(* Logix 5000 AddOnInstructionDefinition export Process_TU3VFDControl_Instance100_101; software revision 24.02 *)

TYPE FI_Data_IN :
STRUCT
   ConnectionFaulted : BOOL;
   RunMode : BOOL;
   Data : INT[6];   // Actual Values
END_STRUCT
END_TYPE

TYPE FI_Data_OUT :
STRUCT
   Data : INT[6];   // Control Data
END_STRUCT
END_TYPE

ADD_ON_INSTRUCTION Process_TU3VFDControl_Instance100_101   (* revision 1.1, vendor NORD Drivesystems, ExecutePrescan *)
// Control block for Nord VFD TU3 Instances 100/101
// Allows for control of one (1) SK 5xxE VFD.
// Revision note:
// Rev 1.1
// Better Ready Start Condition Logic
// Added Inhibited Output
// Added Fault Active Output
// Rev 1.0
VAR_IN_OUT
   FI_Status : _0342:TU3_EIP_DE5BFA94:I:0; {required}   // Input Data Map of VFD
   FI_Control : _0342:TU3_EIP_E8E6FFA2:O:0; {required}   // Output Data Map of VFD
END_VAR
VAR_INPUT
   VFD_Number : SINT := 1;   // Number of VFD to control (1 for Instance 100/101)
   EnableFwd : BOOL; {visible}   // HIGH = Enable CW
   EnableRev : BOOL; {visible}   // HIGH = Enable CCW
   DisableVoltage : BOOL := 1; {visible}   // LOW = No Output Voltage
   QuickStop : BOOL := 1; {visible}   // LOW = Emergency Stop Active
   FaultAckn : BOOL; {visible}   // Error / Fault Acknowledgement on Rising Edge
   ParameterSet : SINT; {visible}   // Parameter Set 1-4, If less than 1 or higher than 4, Set 1 as active
   Activate32BitSetpoint : BOOL; {visible}   // HIGH = Activate 32Bit Setpoint combining Setpoint 2 & 3
   ControlWordBit8_P480_11 : BOOL; {visible}   // Control Word Bit 8 Function set in P480[11]
   ControlWordBit9_P480_12 : BOOL; {visible}   // Control Word Bit 9 Function set in P480[12]
END_VAR
VAR_OUTPUT
   ControlWord : ALIAS FOR Control_Word; {access Read Only, visible}   // Control Word Read Only Version
END_VAR
VAR_INPUT
   Setpoint1 : INT; {visible}   // Setpoint 1 Function set in P546
   Setpoint2 : INT; {visible}   // Setpoint 2 Function set in P547, deactivated if "PositioningActiveBit" is set
   Setpoint3 : INT; {visible}   // Setpoint 3 Function set in P548, deactivated if "PositioningActiveBitt" is set
   Setpoint4 : INT;   // Setpoint 4 Only available in SK 54xE
   Setpoint5 : INT;   // Setpoint 5 Only available in SK 54xE
   Setpoint2_3_32 : DINT; {visible}   // 32 Bit Setpoint 2 & 3 combined for positioning
END_VAR
VAR_OUTPUT
   StatusWord : INT; {access Read Only, visible}   // Status Word
        .0   // Ready to Start
        .1   // Ready for Operation
        .2   // Operation Enabled
        .3   // Fault
        .4   // Voltage Enabled
        .5   // No Emergency Stop
        .6   // Starting Disabled
        .7   // Warning Active
        .8   // Setpoint Reached
        .9   // Bus Controller Active
        .10   // Function P481[9]
        .11   // Rotation Right Active
        .12   // Rotation Left Active
        .13   // Function P481[10]
        .14   // Parameter Set Bit 0
        .15   // Parameter Set Bit 1
   ActiveParameterSet : SINT; {access None, visible}   // Displays Active Parameter set
   CommunicationOK : BOOL; {access Read Only, visible}   // HIGH = Communication is OK
   ReadyToStart : BOOL; {access None, visible}   // HIGH = Drive Ready to Start
   VFD_Enabled : BOOL; {access None, visible}   // HIGH = VFD is Enabled
   Inhibited : BOOL; {access Read Only, visible}   // VFD is Inhibited
   Warning : BOOL; {access None, visible}   // HIGH = Drive has a warning
   Faulted : BOOL; {access None, visible}   // HIGH = Drive Faulted
   FaultActive : BOOL; {access Read Only, visible}   // Fault Conditions are Currently Active
   StatusWordBit10_P481_9 : BOOL; {access None, visible}   // Status Word Bit 10 Function set in P481[9]
   StatusWordBit13_P481_10 : BOOL; {access None, visible}   // Status Word Bit 13 Function set in P481[10]
   ActualValue1 : INT; {access None, visible}   // Actual Value 1 Function set in P543
   ActualValue2 : INT; {access None, visible}   // Actual Value 2 Function set in P544
   ActualValue3 : INT; {access None, visible}   // Actual Value 3 Function set in P545
   ActualValue4 : INT; {access None}   // Actual Value 4 Function only available in SK 54xE
   ActualValue5 : INT; {access None}   // Actual Value 5 Function only available in SK 54xE
   ActualValue2_3_32 : DINT; {access None, visible}   // 32 Bit Actual Value 2 & 3 Combined for Positioning
END_VAR
VAR
   Index : INT; {access None}   // Index of process data based on VFD number
   Control_Word : INT; {access Read Only}   // Control Word
        .0   // Enable Operation
        .1   // Disable Voltage (Low level disables voltage and stops VFD)
        .2   // Emergency Stop (Low level activates ESTOP and stops VFD)
        .3   // Ready for Operation
        .4   // Enable Pulses
        .5   // Enable Ramp
        .6   // Enable Setpoint
        .7   // Error Acknowledge
        .8   // Function P480[11]
        .9   // Function P480[12]
        .10   // Control Data Valid
        .11   // Rotation Direction Right
        .12   // Rotation Direction Left
        .13   // Reserved
        .14   // Parameter Set Bit 0
        .15   // Parameter Set Bit 1
   Control : FI_Data_OUT; {access None}
   Status : FI_Data_IN; {access None}
   LowWordOf32BitSetpoint : DINT; {access None}
   HighWordOf32BitSetpoint : DINT; {access None}
   Temporary_Variable_32BitSepoint : DINT; {access None}
END_VAR

ROUTINE Logic   (* ladder *)
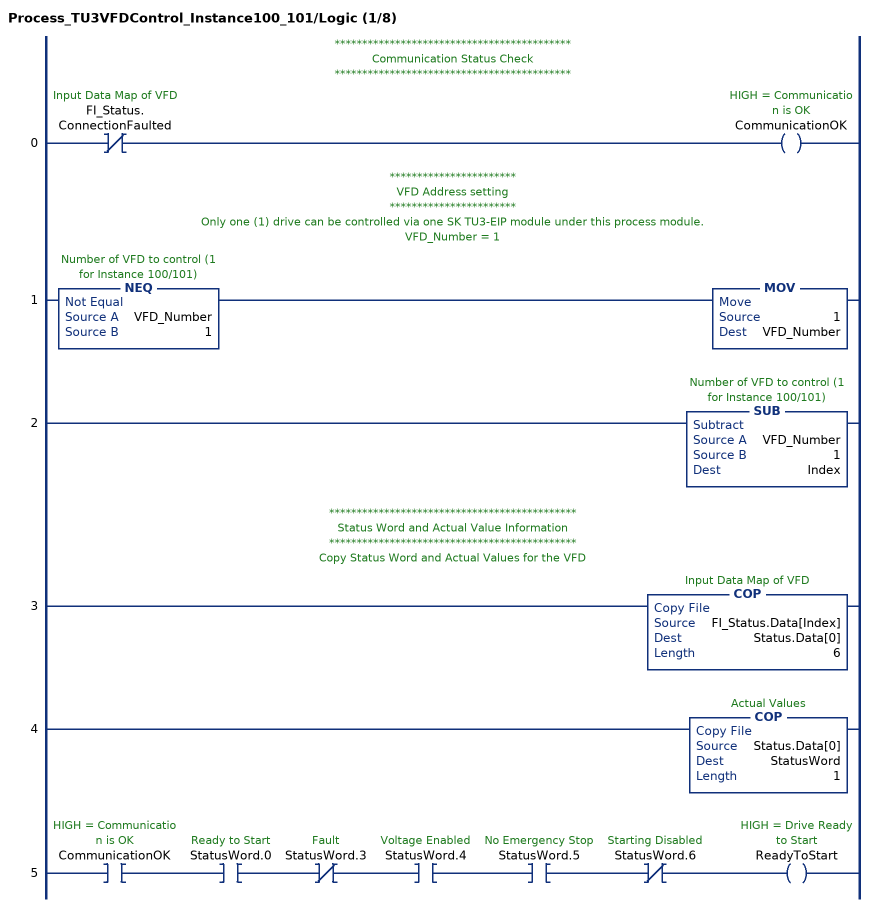
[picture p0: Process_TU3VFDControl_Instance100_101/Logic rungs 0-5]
   // *******************************************
   // Communication Status Check
   // *******************************************
   0: XIO(FI_Status.ConnectionFaulted)OTE(CommunicationOK);
   // ***********************
   // VFD Address setting
   // ***********************
   // Only one (1) drive can be controlled via one SK TU3-EIP module under this process module.
   // VFD_Number = 1
   1: NEQ(VFD_Number,1)MOV(1,VFD_Number);
   2: SUB(VFD_Number,1,Index);
   // *********************************************
   // Status Word and Actual Value Information
   // *********************************************
   // Copy Status Word and Actual Values for the VFD
   3: COP(FI_Status.Data[Index],Status.Data[0],6);
   4: COP(Status.Data[0],StatusWord,1);
   5: XIC(CommunicationOK)XIC(StatusWord.0)XIO(StatusWord.3)XIC(StatusWord.4)XIC(StatusWord.5)XIO(StatusWord.6)OTE(ReadyToStart);
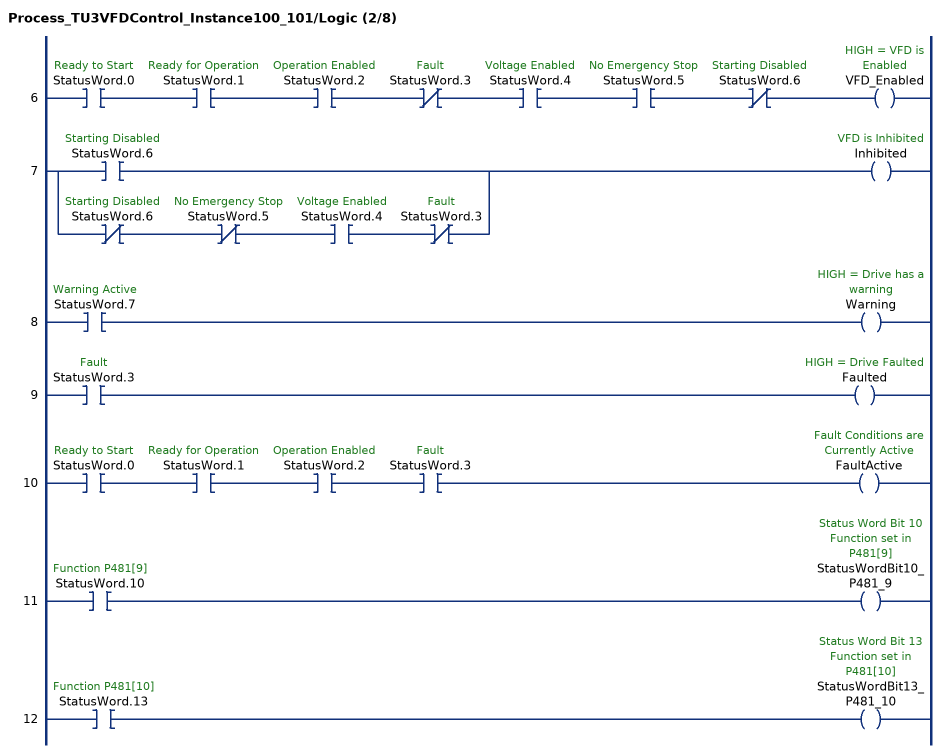
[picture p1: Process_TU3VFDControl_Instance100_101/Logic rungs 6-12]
   6: XIC(StatusWord.0)XIC(StatusWord.1)XIC(StatusWord.2)XIO(StatusWord.3)XIC(StatusWord.4)XIC(StatusWord.5)XIO(StatusWord.6)OTE(VFD_Enabled);
   7: [XIC(StatusWord.6) ,XIO(StatusWord.6) XIO(StatusWord.5) XIC(StatusWord.4) XIO(StatusWord.3) ]OTE(Inhibited);
   8: XIC(StatusWord.7)OTE(Warning);
   9: XIC(StatusWord.3)OTE(Faulted);
   10: XIC(StatusWord.0)XIC(StatusWord.1)XIC(StatusWord.2)XIC(StatusWord.3)OTE(FaultActive);
   11: XIC(StatusWord.10)OTE(StatusWordBit10_P481_9);
   12: XIC(StatusWord.13)OTE(StatusWordBit13_P481_10);
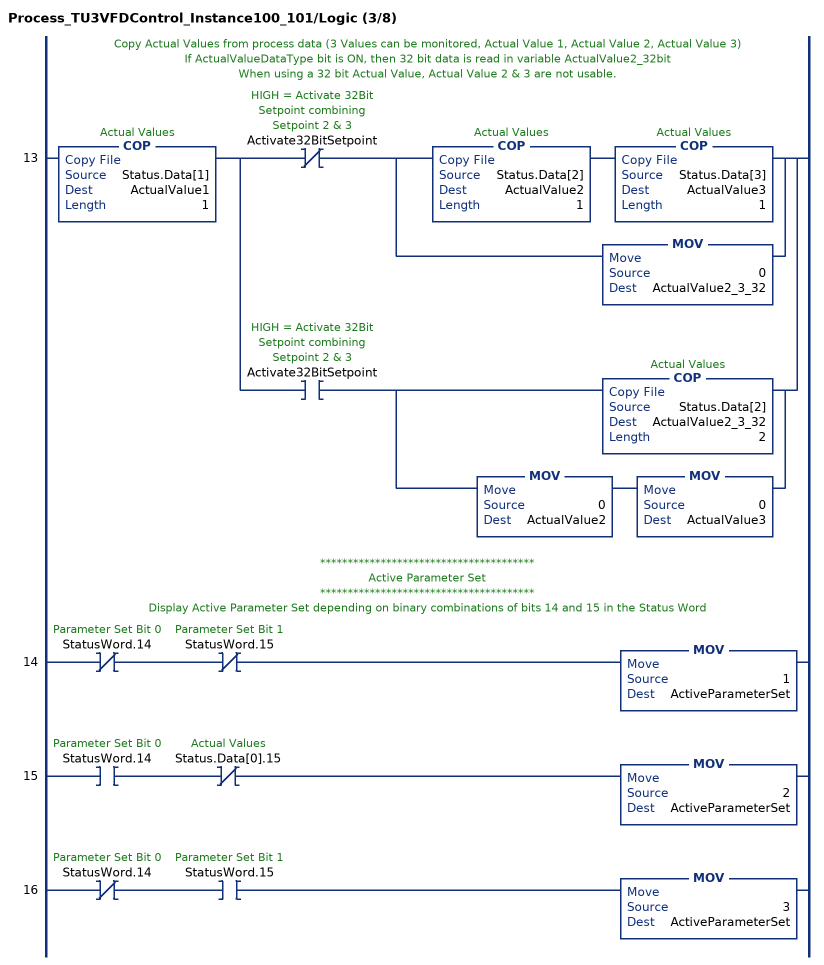
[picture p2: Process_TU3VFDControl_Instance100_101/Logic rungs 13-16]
   // Copy Actual Values from process data (3 Values can be monitored, Actual Value 1, Actual Value 2, Actual Value 3)
   // If ActualValueDataType bit is ON, then 32 bit data is read in variable ActualValue2_32bit
   // When using a 32 bit Actual Value, Actual Value 2 & 3 are not usable.
   13: COP(Status.Data[1],ActualValue1,1)[XIO(Activate32BitSetpoint) [COP(Status.Data[2],ActualValue2,1) COP(Status.Data[3],ActualValue3,1) ,MOV(0,ActualValue2_3_32) ] ,XIC(Activate32BitSetpoint) [COP(Status.Data[2],ActualValue2_3_32,2) ,MOV(0,ActualValue2) MOV(0,ActualValue3) ] ];
   // ***************************************
   // Active Parameter Set
   // ***************************************
   // Display Active Parameter Set depending on binary combinations of bits 14 and 15 in the Status Word
   14: XIO(StatusWord.14)XIO(StatusWord.15)MOV(1,ActiveParameterSet);
   15: XIC(StatusWord.14)XIO(Status.Data[0].15)MOV(2,ActiveParameterSet);
   16: XIO(StatusWord.14)XIC(StatusWord.15)MOV(3,ActiveParameterSet);
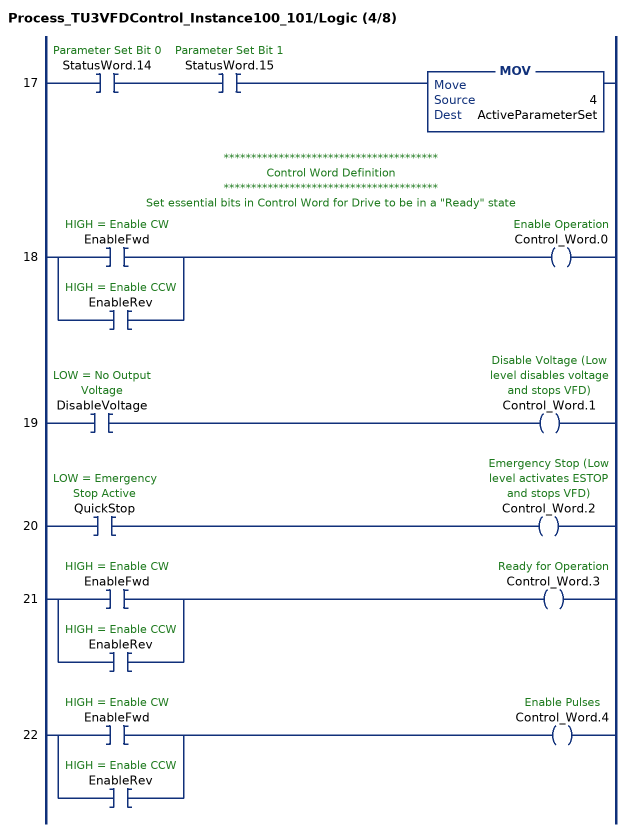
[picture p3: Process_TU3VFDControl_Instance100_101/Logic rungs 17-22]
   17: XIC(StatusWord.14)XIC(StatusWord.15)MOV(4,ActiveParameterSet);
   // ***************************************
   // Control Word Definition
   // ***************************************
   // Set essential bits in Control Word for Drive to be in a "Ready" state
   18: [XIC(EnableFwd) ,XIC(EnableRev) ]OTE(Control_Word.0);
   19: XIC(DisableVoltage)OTE(Control_Word.1);
   20: XIC(QuickStop)OTE(Control_Word.2);
   21: [XIC(EnableFwd) ,XIC(EnableRev) ]OTE(Control_Word.3);
   22: [XIC(EnableFwd) ,XIC(EnableRev) ]OTE(Control_Word.4);
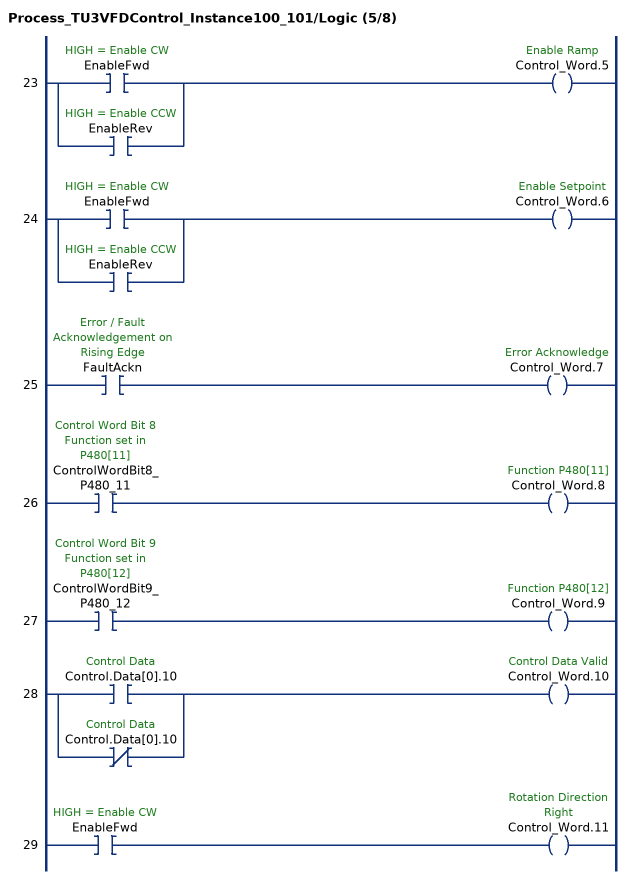
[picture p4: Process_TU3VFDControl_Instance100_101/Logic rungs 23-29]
   23: [XIC(EnableFwd) ,XIC(EnableRev) ]OTE(Control_Word.5);
   24: [XIC(EnableFwd) ,XIC(EnableRev) ]OTE(Control_Word.6);
   25: XIC(FaultAckn)OTE(Control_Word.7);
   26: XIC(ControlWordBit8_P480_11)OTE(Control_Word.8);
   27: XIC(ControlWordBit9_P480_12)OTE(Control_Word.9);
   28: [XIC(Control.Data[0].10) ,XIO(Control.Data[0].10) ]OTE(Control_Word.10);
   29: XIC(EnableFwd)OTE(Control_Word.11);
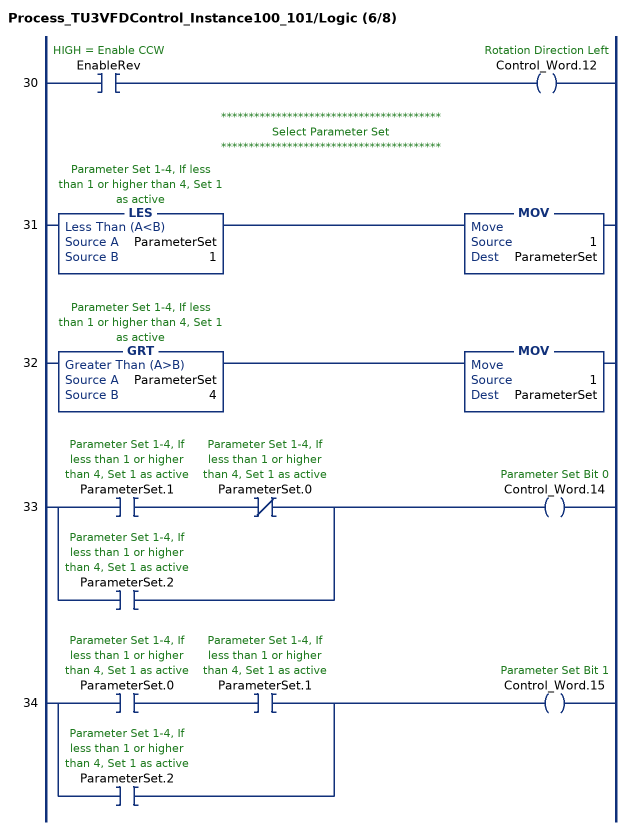
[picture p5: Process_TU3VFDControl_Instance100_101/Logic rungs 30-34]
   30: XIC(EnableRev)OTE(Control_Word.12);
   // ****************************************
   // Select Parameter Set
   // ****************************************
   31: LES(ParameterSet,1)MOV(1,ParameterSet);
   32: GRT(ParameterSet,4)MOV(1,ParameterSet);
   33: [XIC(ParameterSet.1) XIO(ParameterSet.0) ,XIC(ParameterSet.2) ]OTE(Control_Word.14);
   34: [XIC(ParameterSet.0) XIC(ParameterSet.1) ,XIC(ParameterSet.2) ]OTE(Control_Word.15);
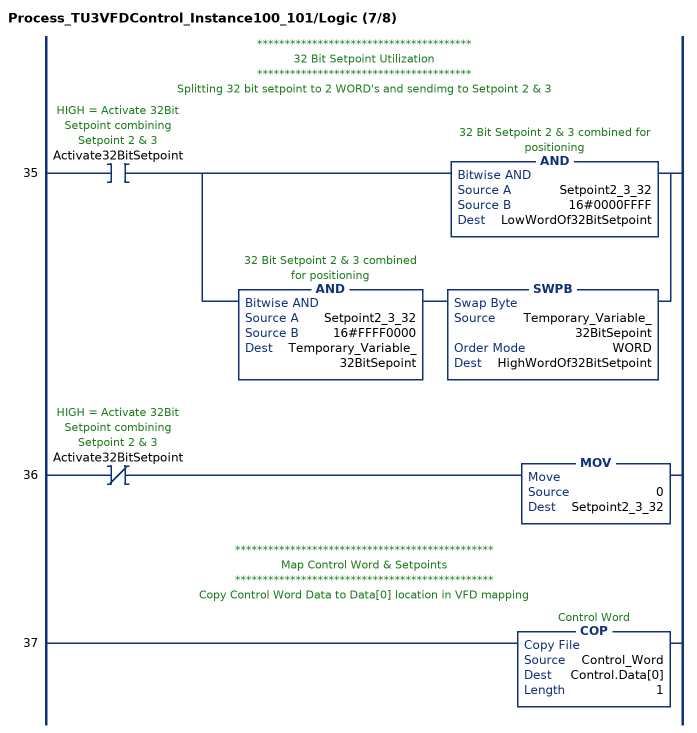
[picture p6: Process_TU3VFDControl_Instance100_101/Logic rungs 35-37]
   // ***************************************
   // 32 Bit Setpoint Utilization
   // ***************************************
   // Splitting 32 bit setpoint to 2 WORD's and sendimg to Setpoint 2 & 3
   35: XIC(Activate32BitSetpoint)[AND(Setpoint2_3_32,16#0000FFFF,LowWordOf32BitSetpoint) ,AND(Setpoint2_3_32,16#FFFF0000,Temporary_Variable_32BitSepoint) SWPB(Temporary_Variable_32BitSepoint,WORD,HighWordOf32BitSetpoint) ];
   36: XIO(Activate32BitSetpoint)MOV(0,Setpoint2_3_32);
   // ***********************************************
   // Map Control Word & Setpoints
   // ***********************************************
   // Copy Control Word Data to Data[0] location in VFD mapping
   37: COP(Control_Word,Control.Data[0],1);
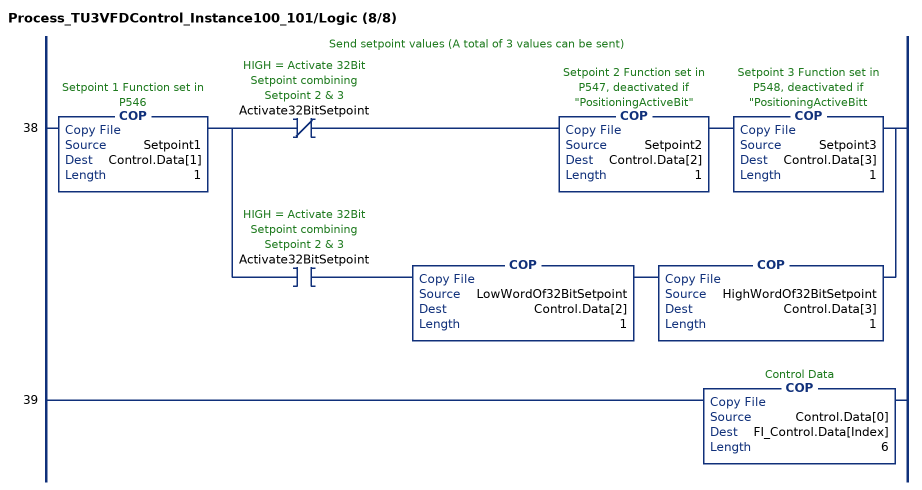
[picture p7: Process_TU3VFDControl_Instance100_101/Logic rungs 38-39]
   // Send setpoint values (A total of 3 values can be sent)
   38: COP(Setpoint1,Control.Data[1],1)[XIO(Activate32BitSetpoint) COP(Setpoint2,Control.Data[2],1) COP(Setpoint3,Control.Data[3],1) ,XIC(Activate32BitSetpoint) COP(LowWordOf32BitSetpoint,Control.Data[2],1) COP(HighWordOf32BitSetpoint,Control.Data[3],1) ];
   39: COP(Control.Data[0],FI_Control.Data[Index],6);
END_ROUTINE

ROUTINE Prescan   (* ladder *)
// Executed prior to first scan of AOI
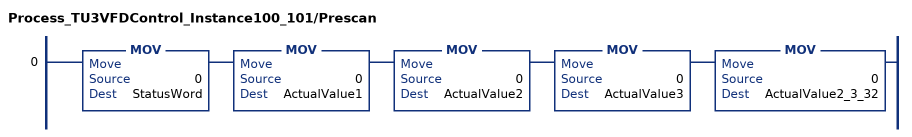
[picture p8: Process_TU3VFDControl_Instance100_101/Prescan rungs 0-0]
   0: MOV(0,StatusWord)MOV(0,ActualValue1)MOV(0,ActualValue2)MOV(0,ActualValue3)MOV(0,ActualValue2_3_32);
END_ROUTINE
END_ADD_ON_INSTRUCTION
